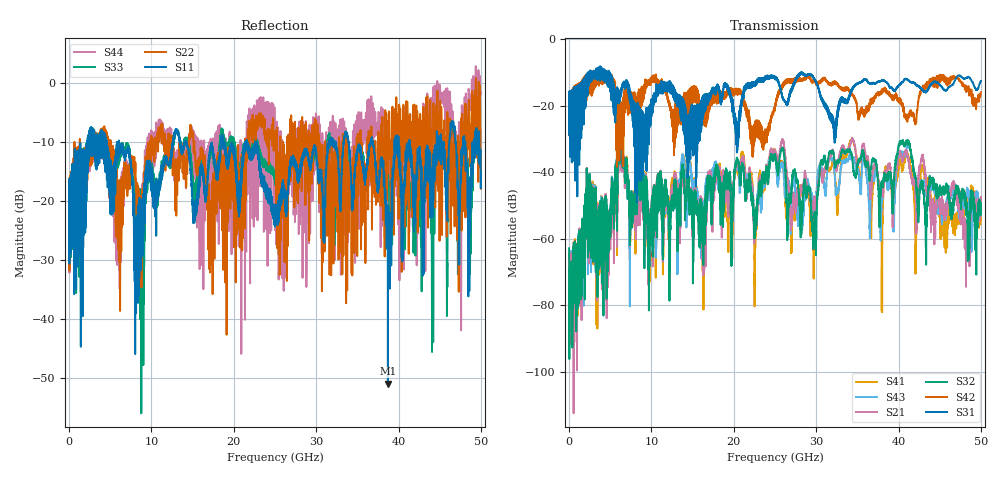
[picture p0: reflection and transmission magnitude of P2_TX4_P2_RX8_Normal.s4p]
!Keysight Technologies,N5225B,MY57041031,A.13.20.10
!Date: Friday, May 31, 2019 11:39:31
!Correction: S11(Full 4 Port(1,2,3,4))
!S12(Full 4 Port(1,2,3,4))
!S13(Full 4 Port(1,2,3,4))
!S14(Full 4 Port(1,2,3,4))
!S21(Full 4 Port(1,2,3,4))
!S22(Full 4 Port(1,2,3,4))
!S23(Full 4 Port(1,2,3,4))
!S24(Full 4 Port(1,2,3,4))
!S31(Full 4 Port(1,2,3,4))
!S32(Full 4 Port(1,2,3,4))
!S33(Full 4 Port(1,2,3,4))
!S34(Full 4 Port(1,2,3,4))
!S41(Full 4 Port(1,2,3,4))
!S42(Full 4 Port(1,2,3,4))
!S43(Full 4 Port(1,2,3,4))
!S44(Full 4 Port(1,2,3,4))
!S4P File: Measurements: <S11,S12,S13,S14>,
!<S21,S22,S23,S24>,
!<S31,S32,S33,S34>,
!<S41,S42,S43,S44>:
# Hz S  dB  R 50.0
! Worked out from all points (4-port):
!   5000 points, 10 MHz to 50 GHz, reference 50 ohm
!   strongest paths, dB at 10 MHz, 12.51 GHz, 25.01 GHz, 37.51 GHz, 50 GHz:
!     S31: -19.2, -14.3, -11.3, -12.8, -12.5
!     S42: -19.6, -21.6, -19.9, -16.5, -16.0
!     S32: -62.9, -47.0, -35.0, -43.4, -50.0
!     S21: -72.0, -44.6, -33.9, -42.0, -48.6
!     S43: -80.3, -44.2, -35.0, -42.7, -51.5
!     S41: -66.3, -42.4, -33.8, -41.6, -53.3
!   lowest |S11| = -50.9 dB at 38.71 GHz (marker M1), VSWR 1.01, Z = 49.8 - j0.149 ohm
!   |S11| at or under -10 dB: 6.073 GHz to 12.61 GHz (6.542 GHz wide, 70 % of centre); 14.21 GHz to 18.43 GHz (4.227 GHz wide, 25.9 % of centre); 22.71 GHz to 31.52 GHz (8.806 GHz wide, 32.5 % of centre)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
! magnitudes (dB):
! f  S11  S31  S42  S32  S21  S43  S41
! 10 MHz  -19.0  -19.2  -19.6  -62.9  -72.0  -80.3  -66.3
! 6.25 GHz  -11.1  -17.3  -29.6  -31.7  -32.8  -31.2  -32.0
! 9.82 GHz  -14.1  -20.2  -12.4  -58.7  -56.0  -56.9  -58.1
! 13.79 GHz  -11.3  -19.4  -21.5  -38.0  -39.0  -34.6  -34.7
! 22.62 GHz  -10.5  -13.9  -24.9  -53.1  -53.3  -53.5  -59.6
! 38.71 GHz  -50.9  -13.5  -16.4  -41.9  -38.6  -44.3  -40.1
! 50 GHz  -15.1  -12.5  -16.0  -50.0  -48.6  -51.5  -53.3
